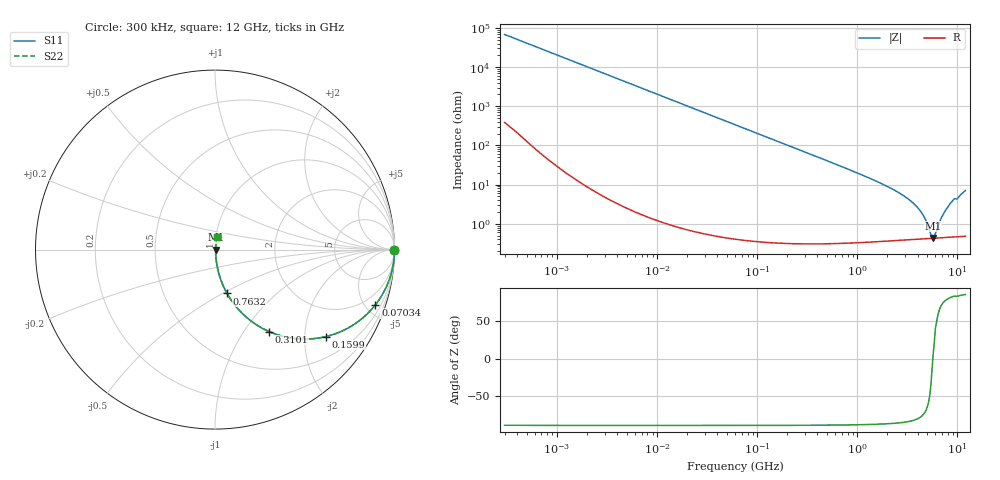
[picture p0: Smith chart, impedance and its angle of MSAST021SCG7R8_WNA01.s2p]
! MSAST021SCG7R8_WNA01  S-PARAMETER MODEL  ( General Type )
! Model Generated by TAIYO YUDEN Corporation (http://www.ty-top.com)
! Version 2.0
! TAIYO YUDEN Control No. 181101
! Copyright(c) 2015 TAIYO YUDEN CO.,LTD. All Rights Reserved.
! Product Description (link to TY-COMPAS)
! https://ds.yuden.co.jp/TYCOMPAS/or/detail?pn=MSAST021SCG7R8CWNA01&u=M
! Products Name : Multilayer Ceramic Capacitors
! Characteristics :
!  Capacitance : 7.8 pF , Rated Voltage : 25V , TCC : CG / C0G
!  Case Size : 0.25 x 0.125 / 0.0098 x 0.0049 [mm/inch] , Thickness : 0.125 / 0.0049 [mm/inch]
!  (Conditions: Temperature = 25 degC , DC Bias Current/Voltage = 0A / 0V)
! External Node Assignments :
!  1  o---| |---o  2
! GND o---------o GND
! Frequency Range : 0.3MHz  -  12000MHz  [ 401 STEP ]
# MHz S RI R 50
! Freq[MHz].  S11 Real  S11 Imag  S21 Real  S21 Imag  S12 Real  S12 Imag  S22 Real  S22 Imag
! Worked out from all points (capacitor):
!   401 points, 300 kHz to 12 GHz, reference 50 ohm
!   read as one part in series: C = 7.8 pF near 316.3 kHz
!   lowest |Z| = 431 mohm at 5.715 GHz (marker M1)
!   series resonance near 5.679 GHz, so ESL is about 100 pH
!   S11 on the Smith chart (normalised r, x): 300 kHz: open; 70.34 MHz: 1.01, -5.80; 159.9 MHz: 1.01, -2.55; 310.1 MHz: 1.01, -1.31; 763.2 MHz: 1.01, -0.52; 12 GHz: 1.01, +0.14
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0.3  1 -0.00147  1.05e-05 0.00147  1.05e-05 0.00147  1 -0.00147
1.769972  0.9999 -0.00867  8.32e-05 0.00867  8.32e-05 0.00867  0.9999 -0.00867
10.44266  0.9974 -0.051  0.00264 0.051  0.00264 0.051  0.9974 -0.051
27.10171  0.9826 -0.1305  0.0174 0.1305  0.0174 0.1305  0.9826 -0.1305
60  0.9201 -0.2705  0.0799 0.2705  0.0799 0.2705  0.9201 -0.2705
70.33673  0.8934 -0.3079  0.1066 0.3079  0.1066 0.3079  0.8934 -0.3079
104.6549  0.7912 -0.4056  0.2088 0.4056  0.2088 0.4056  0.7912 -0.4056
159.8975  0.6189 -0.4844  0.3811 0.4844  0.3811 0.4844  0.6189 -0.4844
310.0777  0.3018 -0.4567  0.6982 0.4567  0.6982 0.4567  0.3018 -0.4567
353.9943  0.2491 -0.4298  0.7509 0.4298  0.7509 0.4298  0.2491 -0.4298
763.2128  0.0671 -0.2441  0.9329 0.2441  0.9329 0.2441  0.0671 -0.2441
2088.533  0.0106 -0.0832  0.9894 0.0832  0.9894 0.0832  0.0106 -0.0832
3026.31  0.00614 -0.0477  0.9939 0.0477  0.9939 0.0477  0.00614 -0.0477
3944.255  0.00472 -0.0264  0.9953 0.0264  0.9953 0.0264  0.00472 -0.0264
4623.766  0.00434 -0.0146  0.9957 0.0146  0.9957 0.0146  0.00434 -0.0146
5420.343  0.00425 -0.00314  0.9958 0.00314  0.9958 0.00314  0.00425 -0.00314
5715.274  0.00427 0.000403  0.9957 -0.000403  0.9957 -0.000403  0.00427 0.000403
6026.253  0.00432 0.00373  0.9957 -0.00373  0.9957 -0.00373  0.00432 0.00373
7064.448  0.00465 0.0152  0.9953 -0.0152  0.9953 -0.0152  0.00465 0.0152
8064.993  0.00523 0.0267  0.9948 -0.0267  0.9948 -0.0267  0.00523 0.0267
8966.534  0.00604 0.0382  0.994 -0.0382  0.994 -0.0382  0.00604 0.0382
12000  0.00967 0.0696  0.9903 -0.0696  0.9903 -0.0696  0.00967 0.0696
